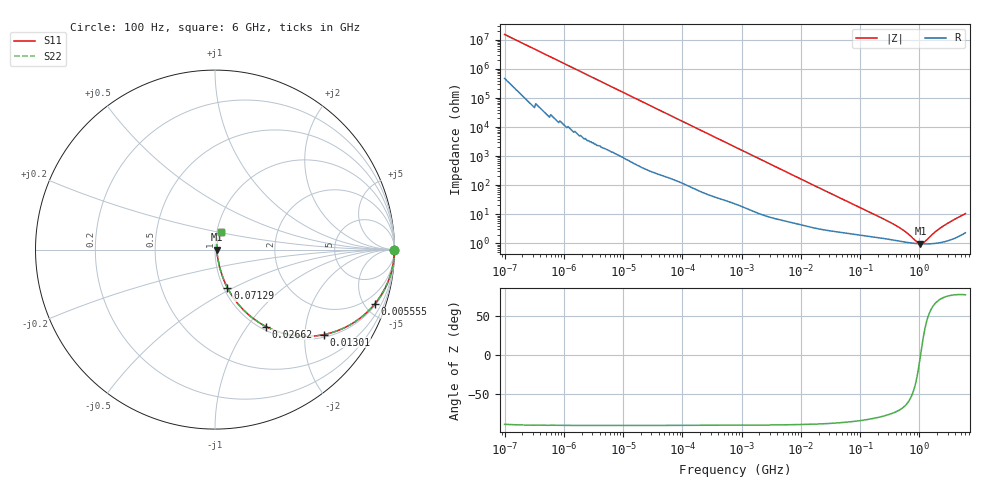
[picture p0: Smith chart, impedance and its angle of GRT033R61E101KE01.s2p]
!Murata Part Number: GRT033R61E101KE01
!These Parameters are Measured in Series Mode Connection
!Data Generated on Jun 19, 2026
!  o--ll--o
!Port1  Port2
!  o------o
!Operation Temp=25[degC], DC Bias Voltage=0[V]
!Freq. Start=100[Hz] Stop=6[GHz] 401[Steps]
# Hz S RI R 50
!Freq.(Hz) S11(Real) S11(Imag) S21(Real) S21(Imag) S12(Real) S12(Imag) S22(Real) S22(Imag)
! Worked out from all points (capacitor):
!   401 points, 100 Hz to 6 GHz, reference 50 ohm
!   read as one part in series: C = 103 pF near 109 Hz
!   lowest |Z| = 957 mohm at 1.047 GHz (marker M1)
!   series resonance near 1.05 GHz, so ESL is about 220 pH
!   S11 on the Smith chart (normalised r, x): 100 Hz: open; 5.555 MHz: 1.12, -5.81; 13.01 MHz: 1.08, -2.51; 26.62 MHz: 1.06, -1.23; 71.29 MHz: 1.04, -0.47; 6 GHz: 1.05, +0.20
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100  1 -6.5e-06  2e-07 6.5e-06  2e-07 6.5e-06  1 -6.5e-06
1404  1 -9.03e-05  6e-07 9.03e-05  6e-07 9.03e-05  1 -9.03e-05
2008  1 -0.000129  8e-07 0.000129  8e-07 0.000129  1 -0.000129
40335  1 -0.00257  2.2e-05 0.00257  2.2e-05 0.00257  1 -0.00257
774597  0.9971 -0.0484  0.00289 0.0484  0.00289 0.0484  0.9971 -0.0484
2268635  0.9787 -0.138  0.0213 0.138  0.0213 0.138  0.9787 -0.138
5554849  0.8895 -0.3038  0.1105 0.3038  0.1105 0.3038  0.8895 -0.3038
8311524  0.7863 -0.3979  0.2137 0.3979  0.2137 0.3979  0.7863 -0.3979
1.300572e7  0.608 -0.4733  0.392 0.4733  0.392 0.4733  0.608 -0.4733
1.555665e7  0.5238 -0.4831  0.4762 0.4831  0.4762 0.4831  0.5238 -0.4831
2.662322e7  0.285 -0.4292  0.715 0.4292  0.715 0.4292  0.285 -0.4292
4.165952e7  0.1514 -0.3289  0.8486 0.3289  0.8486 0.3289  0.1514 -0.3289
7.129496e7  0.0696 -0.2136  0.9304 0.2136  0.9304 0.2136  0.0696 -0.2136
1.395531e8  0.0307 -0.1153  0.9693 0.1153  0.9693 0.1153  0.0307 -0.1153
3.124326e8  0.0161 -0.0512  0.9839 0.0512  0.9839 0.0512  0.0161 -0.0512
5.346885e8  0.0118 -0.0255  0.9882 0.0255  0.9882 0.0255  0.0118 -0.0255
9.150511e8  0.00967 -0.005  0.9903 0.005  0.9903 0.005  0.00967 -0.005
1.046602e9  0.00948 -0.000112  0.9905 0.000112  0.9905 0.000112  0.00948 -0.000112
1.197065e9  0.00943 0.00481  0.9906 -0.00481  0.9906 -0.00481  0.00943 0.00481
1.791126e9  0.0102 0.0206  0.9898 -0.0206  0.9898 -0.0206  0.0102 0.0206
2.562649e9  0.0124 0.0372  0.9876 -0.0372  0.9876 -0.0372  0.0124 0.0372
6e9  0.0321 0.0967  0.9679 -0.0967  0.9679 -0.0967  0.0321 0.0967
